(* Logix 5000 AddOnInstructionDefinition export AMCI_MA_Run_Blend_Move; software revision 20.05 *)

TYPE AMCI_Motion_Axis_Output_Data :
STRUCT
   Control_Word_0 : INT;
   Control_Word_1 : INT;
   Position_or_Distance : DINT;
   Programmed_Speed : DINT;
   Acceleration : INT;
   Deceleration : INT;
   Output_Word_8 : INT;
   Output_Word_9 : INT;
END_STRUCT
END_TYPE

TYPE AMCI_Motion_Axis_Input_Data :
STRUCT
   Moving_CW : BOOL;
   Moving_CCW : BOOL;
   In_Hold_State : BOOL;
   Stopped : BOOL;
   At_Home : BOOL;
   Accelerating : BOOL;
   Decelerating : BOOL;
   Move_Complete : BOOL;
   Status_Word_0_Bit_8 : BOOL;
   Status_Word_0_Bit_9 : BOOL;
   Position_Invalid : BOOL;
   Input_Error : BOOL;
   Command_Error : BOOL;
   Configuration_Error : BOOL;
   Module_OK : BOOL;
   Mode_Flag : BOOL;
   IN1_Active : BOOL;
   IN2_Active : BOOL;
   IN3_Active : BOOL;
   IN4_Active : BOOL;
   Status_Word_1_Bit_4 : BOOL;
   Status_Word_1_Bit_5 : BOOL;
   Connection_Was_Lost : BOOL;
   Driver_Fault : BOOL;
   Status_Word_1_Bit_8 : BOOL;
   Invalid_Jog_Change : BOOL;
   Status_Word_1_Bit_10 : BOOL;
   Heartbeat_Bit : BOOL;
   Status_Word_1_Bit_12 : BOOL;
   Status_Word_1_Bit_13 : BOOL;
   Stall_Detected : BOOL;
   Drive_Is_Enabled : BOOL;
   Motor_Position : DINT;
   Encoder_Position : DINT;
   Trapped_Encoder_Position : DINT;
   Input_Word_8 : INT;
   Input_Word_9 : INT;
END_STRUCT
END_TYPE

ADD_ON_INSTRUCTION AMCI_MA_Run_Blend_Move   (* revision 1.0, vendor AMCI, ExecuteEnableInFalse *)
// Run Blend Moves for SD and SMD devices.  Will not work with SV integrated servo devices.
// Help:
// MOTION AXIS RUN BLEND MOVE
// This AOI will only work with the SD and SMD motion devices.  The SV motion devices do not support Assembled Moves.
// AXIS INPUT DATA:  Input data from AMCI motion device.   Uses the AMCI_Motion_Axis_Input_Data User Defined Data Type.
// AXIS OUTPUT DATA; Output data from the AOI to the AMCI motion device.   Uses the AMCI_Motion_Axis_Output_Data User Defined Data Type.
// DIRECTION: 0 = CW motion 1 = CCW motion
// EN (Enable) Set when rung is true, Reset when rung is false
// DN (Done) Set when command is sent to the motion device.  Reset when the rung is false.
// ER (Error) Set when a command or input error failed to clear.  Reset when the rung is false.
// IP (In Process) Set when motion is occurring.   Reset when motion stops or the rung goes false.
VAR_IN_OUT
   Axis_Input_Data : AMCI_Motion_Axis_Input_Data; {required}
   Axis_Output_Data : AMCI_Motion_Axis_Output_Data; {required}
END_VAR
VAR_INPUT
   Type_0_for_standard_1_for_indexed : BOOL;
   Direction_0_for_CW_1_for_CCW : BOOL; {required}
END_VAR
VAR_OUTPUT
   EN : BOOL; {access Read Only, visible}
   DN : BOOL; {access Read Only, visible}
   ER : BOOL; {access Read Only, visible}
   IP : BOOL; {access Read Only, visible}
END_VAR
VAR
   command_data_block : INT[10];
        [0]   // Command Bits MSW
        [1]   // Command Bits LSW
        [2]   // Upper Target Position
        [3]   // Lower Target Position
        [4]   // Upper Programmed Speed
        [5]   // Lower Programmed Speed
END_VAR

ROUTINE EnableInFalse   (* ladder *)
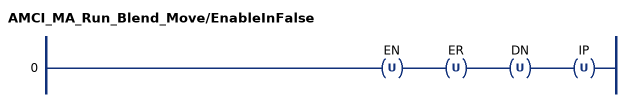
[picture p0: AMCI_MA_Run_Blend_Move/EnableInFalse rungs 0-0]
   0: OTU(EN)OTU(ER)OTU(DN)OTU(IP);
END_ROUTINE

ROUTINE Logic   (* ladder *)
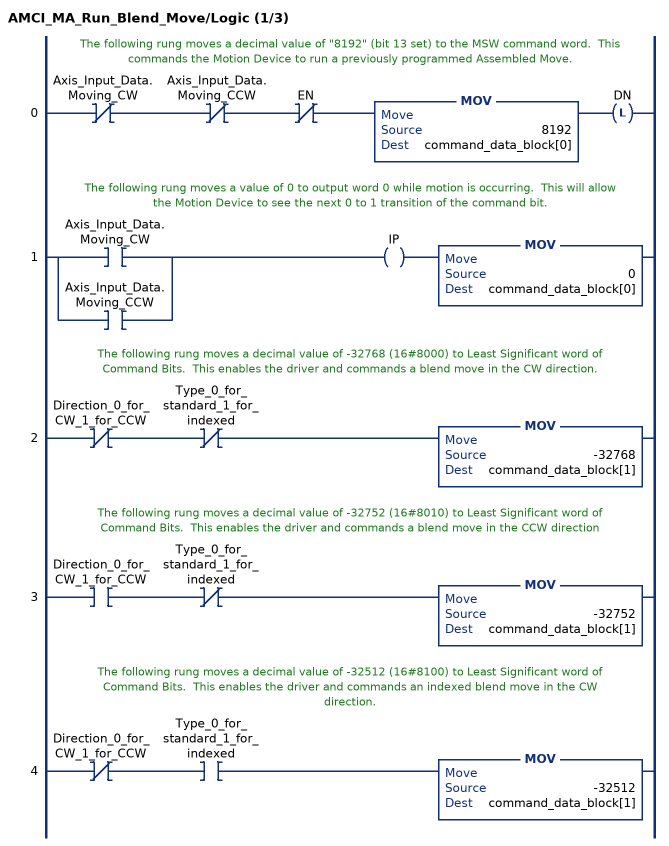
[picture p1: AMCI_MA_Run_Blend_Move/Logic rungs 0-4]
   // The following rung moves a decimal value of "8192" (bit 13 set) to the MSW command word.  This commands the Motion Device to run a previously programmed Assembled Move.
   0: XIO(Axis_Input_Data.Moving_CW)XIO(Axis_Input_Data.Moving_CCW)XIO(EN)MOV(8192,command_data_block[0])OTL(DN);
   // The following rung moves a value of 0 to output word 0 while motion is occurring.  This will allow the Motion Device to see the next 0 to 1 transition of the command bit.
   1: [XIC(Axis_Input_Data.Moving_CW) ,XIC(Axis_Input_Data.Moving_CCW) ]OTE(IP)MOV(0,command_data_block[0]);
   // The following rung moves a decimal value of -32768 (16#8000) to Least Significant word of Command Bits.  This enables the driver and commands a blend move in the CW direction.
   2: XIO(Direction_0_for_CW_1_for_CCW)XIO(Type_0_for_standard_1_for_indexed)MOV(-32768,command_data_block[1]);
   // The following rung moves a decimal value of -32752 (16#8010) to Least Significant word of Command Bits.  This enables the driver and commands a blend move in the CCW direction
   3: XIC(Direction_0_for_CW_1_for_CCW)XIO(Type_0_for_standard_1_for_indexed)MOV(-32752,command_data_block[1]);
   // The following rung moves a decimal value of -32512 (16#8100) to Least Significant word of Command Bits.  This enables the driver and commands an indexed blend move in the CW direction.
   4: XIO(Direction_0_for_CW_1_for_CCW)XIC(Type_0_for_standard_1_for_indexed)MOV(-32512,command_data_block[1]);
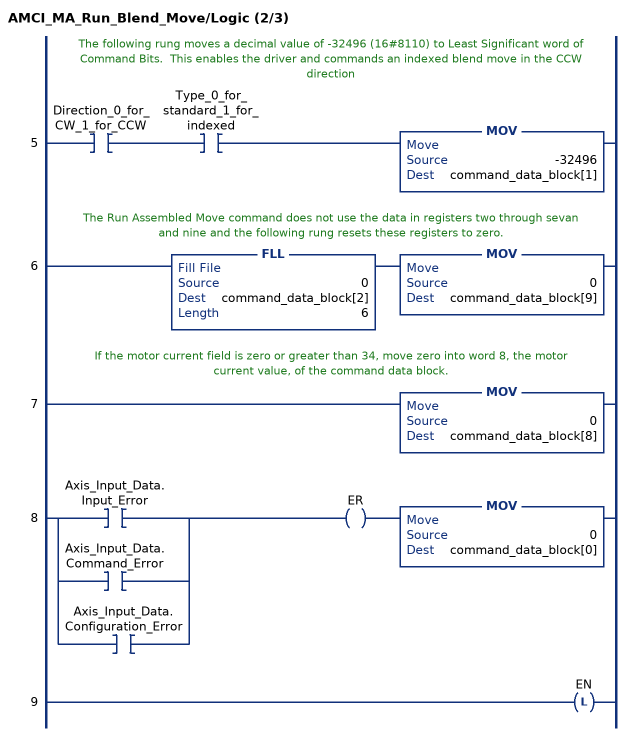
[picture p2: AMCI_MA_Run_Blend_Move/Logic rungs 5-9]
   // The following rung moves a decimal value of -32496 (16#8110) to Least Significant word of Command Bits.  This enables the driver and commands an indexed blend move in the CCW direction
   5: XIC(Direction_0_for_CW_1_for_CCW)XIC(Type_0_for_standard_1_for_indexed)MOV(-32496,command_data_block[1]);
   // The Run Assembled Move command does not use the data in registers two through sevan and nine and the following rung resets these registers to zero.
   6: FLL(0,command_data_block[2],6)MOV(0,command_data_block[9]);
   // If the motor current field is zero or greater than 34, move zero into word 8, the motor current value, of the command data block.
   7: MOV(0,command_data_block[8]);
   8: [XIC(Axis_Input_Data.Input_Error) ,XIC(Axis_Input_Data.Command_Error) ,XIC(Axis_Input_Data.Configuration_Error) ]OTE(ER)MOV(0,command_data_block[0]);
   9: OTL(EN);
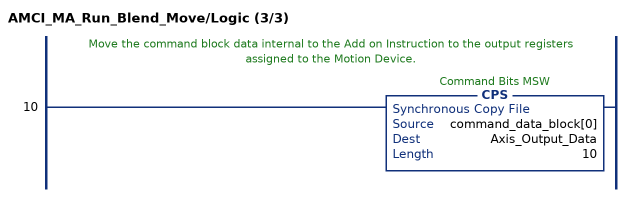
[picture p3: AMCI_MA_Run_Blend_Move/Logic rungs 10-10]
   // Move the command block data internal to the Add on Instruction to the output registers assigned to the Motion Device.
   10: CPS(command_data_block[0],Axis_Output_Data,10);
END_ROUTINE
END_ADD_ON_INSTRUCTION
